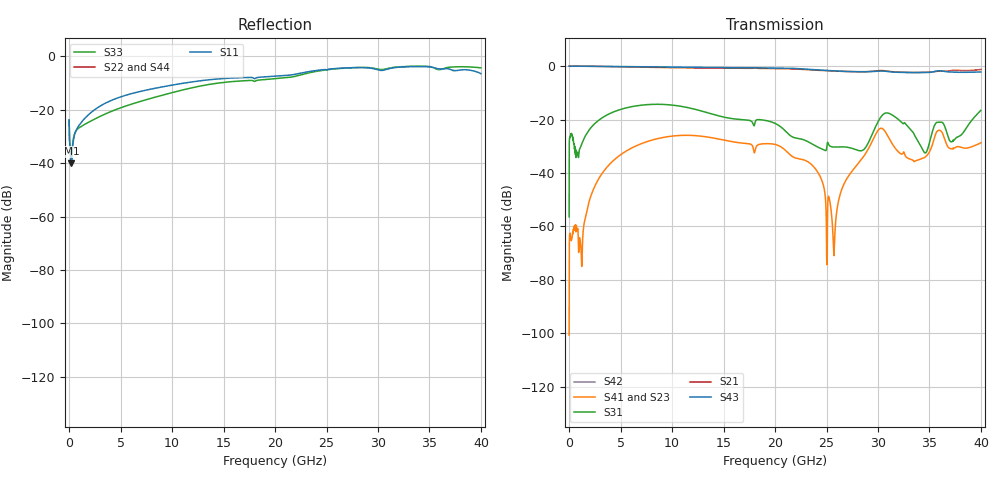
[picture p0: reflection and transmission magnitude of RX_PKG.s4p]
# GHz S MA R 50
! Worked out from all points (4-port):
!   7999 points, 1 MHz to 39.99 GHz, reference 50 ohm
!   strongest paths, dB at 1 MHz, 9.996 GHz, 20 GHz, 30 GHz, 39.99 GHz:
!     S43: 0.0, -0.4, -0.7, -1.8, -2.2
!     S21: 0.0, -0.6, -0.9, -1.7, -1.2
!     S31: -56.4, -14.6, -21.4, -20.9, -16.5
!     S41: -100.7, -26.2, -29.3, -24.1, -28.7
!     S23: -100.7, -26.2, -29.3, -24.1, -28.7
!     S42: -, -, -, -, -
!   lowest |S11| = -40.1 dB at 221 MHz (marker M1), VSWR 1.02, Z = 49 + j0.14 ohm
!   |S11| at or under -10 dB: start of sweep to 11.21 GHz
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0.001  0.06425 -174.1  9.999e-16 -0.4  0.001506 90.5  1e-15 0.3
       0.9979 -0.0  9.978e-16 -177.9  9.184e-06 -0.2  9.981e-16 0.3
       0.001506 90.5  1e-15 0.3  0.06431 -174.1  9.999e-16 -0.4
       9.184e-06 0.2  9.985e-16 0.3  0.9979 -0.0  9.978e-16 -177.9
0.221  0.009883 171.7  9.999e-16 -3.9  0.05484 -2.5  1e-15 -65.7
       0.9984 -0.0  9.981e-16 -171.5  0.0005467 9.4  9.984e-16 -65.8
       0.05484 -2.5  1e-15 -65.7  0.01006 -169.5  9.999e-16 -3.8
       0.0005467 -9.4  9.981e-16 -65.8  0.9984 -0.0  9.984e-16 -171.6
8.691  0.26 12.5  9.885e-16 -6.0  0.193 5.1  9.796e-16 18.3
       0.9451 -0.0  1.024e-15 -168.9  0.04436 174.4  9.551e-16 18.7
       0.193 5.1  9.909e-16 19.5  0.1791 2.1  9.849e-16 -5.1
       0.04436 -174.4  9.8e-16 19.7  0.9637 -0.0  1.036e-15 -170.1
20.496  0.4308 -60.9  9.914e-16 -14.1  0.0731 -45.8  9.573e-16 29.5
        0.8988 -0.0  9.893e-16 -156.2  0.03143 176.6  9.057e-16 25.1
        0.07441 -46.3  9.737e-16 27.7  0.3896 -69.8  9.861e-16 -12.1
        0.03143 -176.6  9.296e-16 24.3  0.9176 -0.0  9.853e-16 -156.5
25.721  0.5882 -84.7  9.997e-16 -20.4  0.0309 2.7  9.341e-16 16.3
        0.8081 -0.0  9.48e-16 -150.5  0.0002866 -80.5  8.667e-16 4.8
        0.03058 4.2  8.926e-16 17.5  0.5795 -88.7  9.947e-16 -18.4
        0.0002866 80.5  8.563e-16 -0.3  0.8144 0.0  9.424e-16 -149.6
30.166  0.547 -117.0  9.567e-16 -35.0  0.103 46.4  1.048e-15 17.2
        0.828 -0.0  8.189e-16 -143.7  0.06739 -0.2  8.04e-16 -6.4
        0.1032 46.3  1.347e-15 19.6  0.5692 -118.2  1.268e-15 -39.6
        0.06739 0.2  3.876e-16 14.2  0.8129 0.0  3.477e-16 -154.8
39.991  0.4731 119.8  9.233e-16 -24.5  0.1488 34.9  1.033e-15 -10.8
        0.8676 -0.0  8.67e-16 -152.6  0.03691 8.1  8.989e-16 -6.1
        0.1488 34.8  1.004e-15 -8.8  0.6083 171.9  8.438e-16 -29.1
        0.03691 -8.1  1e-15 -8.1  0.7788 0.0  8.114e-16 -140.7
